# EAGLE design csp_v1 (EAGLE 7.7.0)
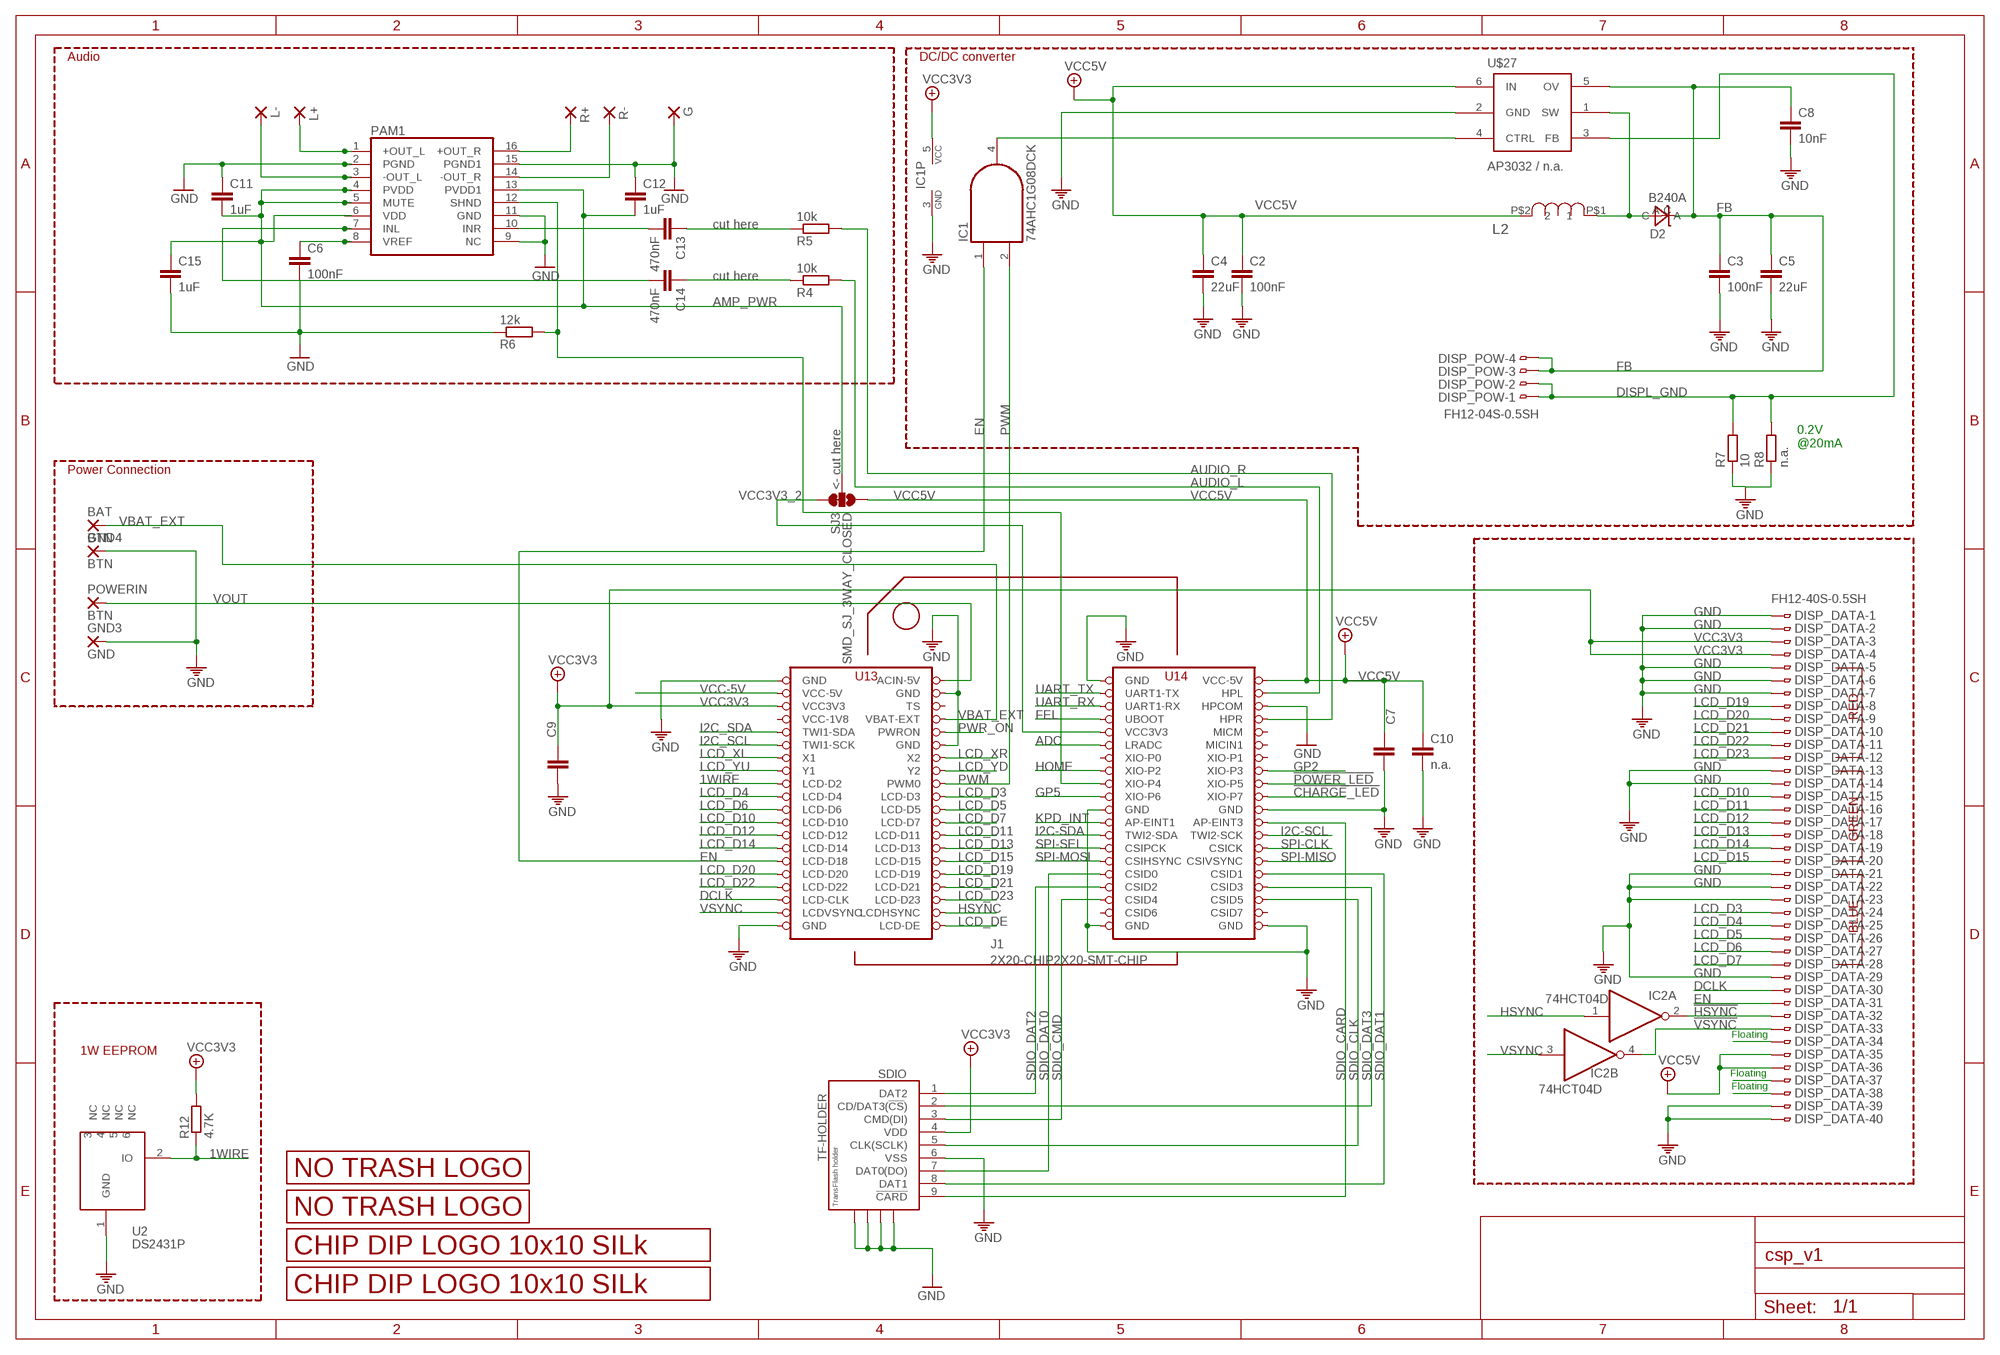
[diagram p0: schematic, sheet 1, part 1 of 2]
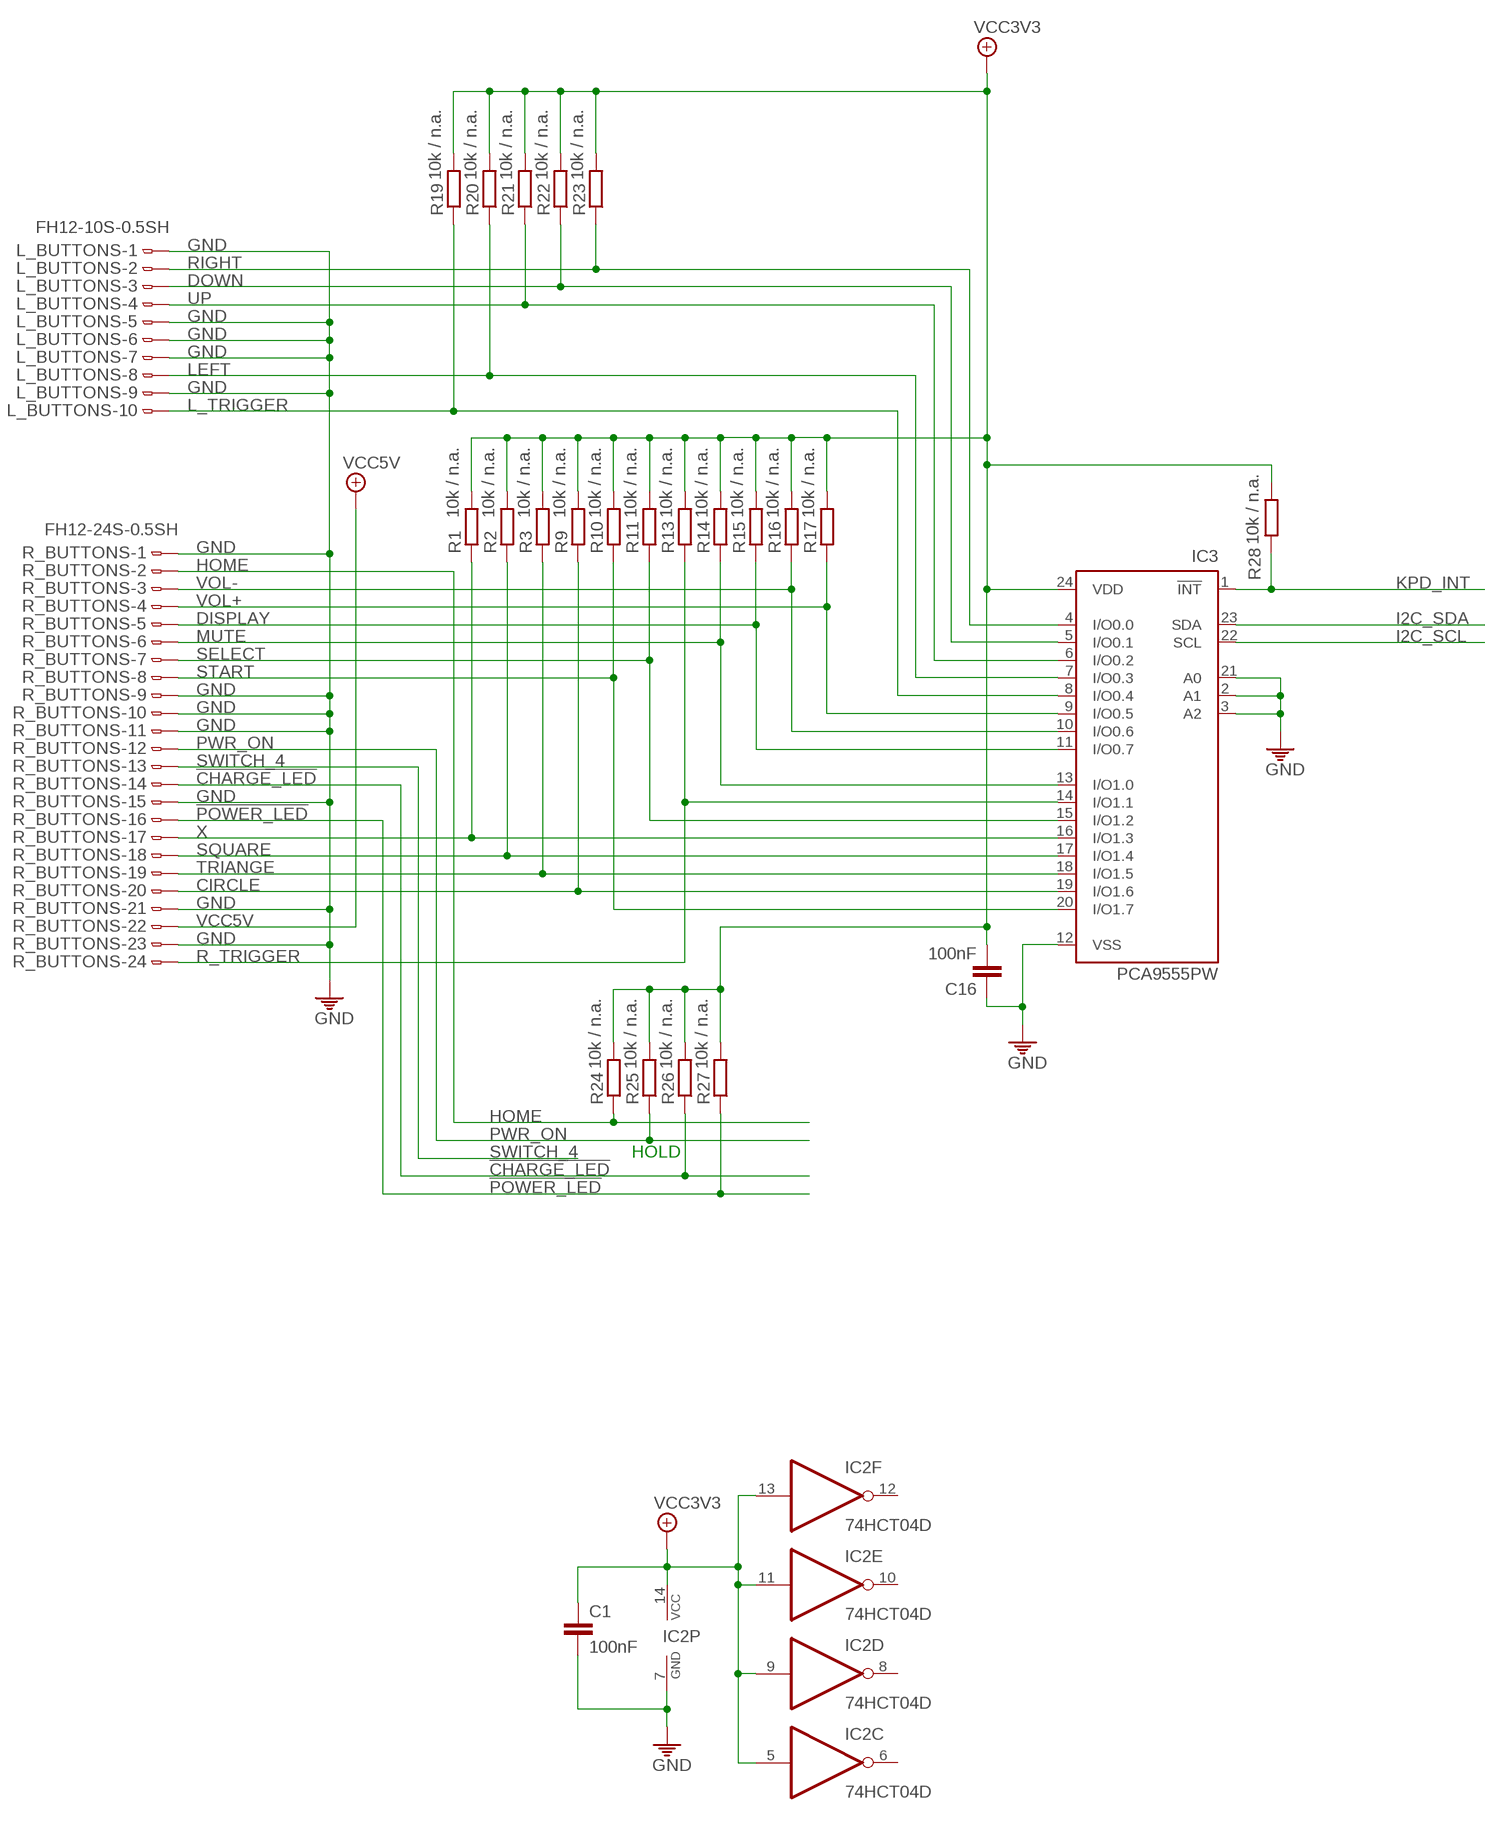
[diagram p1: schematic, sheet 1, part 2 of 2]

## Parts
BAT  BTN  SMD2  [SMD1,27-2,54]
C1  100nF  C-EUC0805  [C0805]
C2  100nF  C-EUC0805  [C0805]
C3  100nF  C-EUC0805  [C0805]
C4  22uF  C-EUC1206  [C1206]
C5  22uF  C-EUC1206  [C1206]
C6  100nF  C-EUC0805  [C0805]
C7  n.a.  C-EUC0805  [C0805]
C8  10nF  C-EUC0805  [C0805]
C9  n.a.  C-EUC0805  [C0805]
C10  n.a.  C-EUC0805  [C0805]
C11  1uF  C-EUC0805  [C0805]
C12  1uF  C-EUC0805  [C0805]
C13  470nF  C-EUC0805  [C0805]
C14  470nF  C-EUC0805  [C0805]
C15  1uF  C-EUC0805  [C0805]
C16  100nF  C-EUC0805  [C0805]
D2  B240A  DIODE_SCHTKY_B240  [DO-214AC]
DISP_DATA  FH12-40S-0.5SH  [FH12-40S-0.5SH]
DISP_POW  FH12-04S-0.5SH  [FH12-04S-0.5SH]
G  1,6/0,8  [1,6/0,8]
GND3  GND  SMD2  [SMD1,27-2,54]
GND4  BTN  SMD2  [SMD1,27-2,54]
IC1  74AHC1G08DCK  [SC70-5]
IC2  74HCT04D  [SO14]
IC3  PCA9555PW  [TSSOP24]
J1  2X20-CHIP2X20-SMT-CHIP  [2XAWHW40_G_SMD_R]
L2  SRN6045-100M  [SRN6045]
L+  1,6/0,8  [1,6/0,8]
L-  1,6/0,8  [1,6/0,8]
L_BUTTONS  FH12-10S-0.5SH  [FH12-10S-0.5SH]
PAM1  PAM8403  [SOP-16]
POWERIN  BTN  SMD2  [SMD1,27-2,54]
R1  10k / n.a.  R-EU_M0805  [M0805]
R2  10k / n.a.  R-EU_M0805  [M0805]
R3  10k / n.a.  R-EU_M0805  [M0805]
R4  10k  R-EU_R0805  [R0805]
R5  10k  R-EU_R0805  [R0805]
R6  12k  R-EU_R0805  [R0805]
R7  10  R-EU_M0805  [M0805]
R8  n.a.  R-EU_M0805  [M0805]
R9  10k / n.a.  R-EU_M0805  [M0805]
R10  10k / n.a.  R-EU_M0805  [M0805]
R11  10k / n.a.  R-EU_M0805  [M0805]
R12  4.7K  R-EU_M0805  [M0805]
R13  10k / n.a.  R-EU_M0805  [M0805]
R14  10k / n.a.  R-EU_M0805  [M0805]
R15  10k / n.a.  R-EU_M0805  [M0805]
R16  10k / n.a.  R-EU_M0805  [M0805]
R17  10k / n.a.  R-EU_M0805  [M0805]
R19  10k / n.a.  R-EU_M0805  [M0805]
R20  10k / n.a.  R-EU_M0805  [M0805]
R21  10k / n.a.  R-EU_M0805  [M0805]
R22  10k / n.a.  R-EU_M0805  [M0805]
R23  10k / n.a.  R-EU_M0805  [M0805]
R24  10k / n.a.  R-EU_M0805  [M0805]
R25  10k / n.a.  R-EU_M0805  [M0805]
R26  10k / n.a.  R-EU_M0805  [M0805]
R27  10k / n.a.  R-EU_M0805  [M0805]
R28  10k / n.a.  R-EU_M0805  [M0805]
R+  1,6/0,8  [1,6/0,8]
R-  1,6/0,8  [1,6/0,8]
R_BUTTONS  FH12-24S-0.5SH  [FH12-24S-0.5SH]
SDIO  TF-HOLDER  [TF-PULL]
SJ3  SMD_SJ_3WAY_CLOSED  [SMD_SJ_3WAY_CLOSED]
U2  DS2431P  [TSOC6]
U$2  LOGO_10X10_SILK  [LOGO2_10X10_SILK]
U$3  LOGO_NO_TRASHROHS  [LOGO_ROHS_SYM]
U$4  LOGO_NO_TRASHNO_TRASH  [LOGO_ROHS_NO_TRASH]
U$5  LOGO_10X10_SILK  [LOGO2_10X10_SILK]
U$27  AP3032 / n.a.  AP3032  [SOT23-6]

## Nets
1WIRE: J1.LCD-D2 R12.1 U2.2(IO)
!CHARGE_LED: J1.XIO-P7 R26.1 R_BUTTONS.14
!HSYNC: DISP_DATA.32 IC2.2(A:O)
!POWER_LED: J1.XIO-P6(XIO-P5) R27.1 R_BUTTONS.16
!VSYNC: DISP_DATA.33 IC2.4(B:O)
ADC: J1.LRADC
AMP_PWR: C11.2 C12.2 C15.1 PAM1.4(PVDD) PAM1.5(MUTE) PAM1.6(VDD) PAM1.13(PVDD1) SJ3.2
AUDIO_L: J1.HPL R4.2
AUDIO_R: J1.HPR R5.2
CIRCLE: IC3.19(I/O1.6) R9.1 R_BUTTONS.20
DCLK: DISP_DATA.30 J1.LCD-CLK
DISPL_GND: DISP_POW.1 DISP_POW.2 R7.2 R8.2 U$27.3(FB)
DISPLAY: IC3.11(I/O0.7) R15.1 R_BUTTONS.5
DOWN: IC3.5(I/O0.1) L_BUTTONS.3 R22.1
EN: DISP_DATA.31 IC1.1(I0) J1.LCD-D18
FB: C3.1 C5.1 C8.1 D2.C DISP_POW.3 DISP_POW.4 U$27.5(OV)
FEL: J1.FEL(UBOOT)
GND: C1.2 C2.2 C3.2 C4.2 C5.2 C6.2 C7.2 C8.2 C9.2 C10.2 C11.1 C12.1 C15.2 C16.1 DISP_DATA.1 DISP_DATA.2 DISP_DATA.5 DISP_DATA.6 DISP_DATA.7 DISP_DATA.13 DISP_DATA.14 DISP_DATA.21 DISP_DATA.22 DISP_DATA.23 DISP_DATA.29 DISP_DATA.39 DISP_DATA.40 G.1(P) GND3.1(P) GND4.1(P) IC1.3(GND) IC2.7(P:GND) IC3.2(A1) IC3.3(A2) IC3.12(VSS) IC3.21(A0) J1.GND@1(GND) J1.GND@2(GND) J1.GND@3(GND) J1.GND@4(GND) J1.GND@5(GND) J1.GND@6(GND) J1.GND@7(GND) J1.GND@8(GND) J1.GND@10(GND) J1.HPCOM L_BUTTONS.1 L_BUTTONS.5 L_BUTTONS.6 L_BUTTONS.7 L_BUTTONS.9 PAM1.2(PGND) PAM1.9(NC) PAM1.11(GND) PAM1.15(PGND1) R6.1 R7.1 R8.1 R_BUTTONS.1 R_BUTTONS.9 R_BUTTONS.10 R_BUTTONS.11 R_BUTTONS.15 R_BUTTONS.21 R_BUTTONS.23 SDIO.6(VSS) SDIO.S1 SDIO.S2 SDIO.S3 SDIO.S4 U2.1(GND) U$27.2(GND)
GP2: J1.XIO-P3
GP3: J1.XIO-P4 PAM1.12(SHND) R6.2
GP5: J1.XIO-P5(XIO-P6)
HOME: J1.XIO-P2 R24.1 R_BUTTONS.2
HSYNC: IC2.1(A:I) J1.LCD-HSYNC(LCDHSYNC)
I2C-SCL: J1.TWI2-SCK
I2C-SDA: J1.TWI2-SDA
I2C_SCL: IC3.22(SCL) J1.TWI1-SCK
I2C_SDA: IC3.23(SDA) J1.TWI1-SDA
INL: C14.2 PAM1.7(INL)
INR: C13.2 PAM1.10(INR)
KPD_INT: IC3.1(!INT) J1.AP-EINT1 R28.1
L+OUT: L+.1(P) PAM1.1(+OUT_L)
L-OUT: L-.1(P) PAM1.3(-OUT_L)
L_TRIGGER: IC3.8(I/O0.4) L_BUTTONS.10 R19.1
LCD_D3: DISP_DATA.24 J1.LCD-D3
LCD_D4: DISP_DATA.25 J1.LCD-D4
LCD_D5: DISP_DATA.26 J1.LCD-D5
LCD_D6: DISP_DATA.27 J1.LCD-D6
LCD_D7: DISP_DATA.28 J1.LCD-D7
LCD_D10: DISP_DATA.15 J1.LCD-D10
LCD_D11: DISP_DATA.16 J1.LCD-D11
LCD_D12: DISP_DATA.17 J1.LCD-D12
LCD_D13: DISP_DATA.18 J1.LCD-D13
LCD_D14: DISP_DATA.19 J1.LCD-D14
LCD_D15: DISP_DATA.20 J1.LCD-D15
LCD_D19: DISP_DATA.8 J1.LCD-D19
LCD_D20: DISP_DATA.9 J1.LCD-D20
LCD_D21: DISP_DATA.10 J1.LCD-D21
LCD_D22: DISP_DATA.11 J1.LCD-D22
LCD_D23: DISP_DATA.12 J1.LCD-D23
LCD_DE: J1.LCD-DE
LCD_XL: J1.X1
LCD_XR: J1.X2
LCD_YD: J1.Y2
LCD_YU: J1.Y1
LEFT: IC3.7(I/O0.3) L_BUTTONS.8 R20.1
MUTE: IC3.13(I/O1.0) R14.1 R_BUTTONS.6
N$1: IC1.4(O) U$27.4(CTRL)
N$9: DISP_DATA.38
N$24: DISP_DATA.37
N$25: DISP_DATA.34
N$38: C6.1 PAM1.8(VREF)
N$41: C14.1 R4.1
N$43: C13.1 R5.1
PWM: IC1.2(I1) J1.PWM0
PWR_ON: J1.PWRON R25.1 R_BUTTONS.12
R+OUT: PAM1.16(+OUT_R) R+.1(P)
R-OUT: PAM1.14(-OUT_R) R-.1(P)
R_TRIGGER: IC3.14(I/O1.1) R13.1 R_BUTTONS.24
RIGHT: IC3.4(I/O0.0) L_BUTTONS.2 R23.1
SDIO_CARD: J1.AP-EINT3 SDIO.9(!CARD)
SDIO_CLK: J1.CSID5 SDIO.5(CLK(SCLK))
SDIO_CMD: J1.CISD4(CSID4) SDIO.3(CMD(DI))
SDIO_DAT0: J1.CSID0 SDIO.7(DAT0(DO))
SDIO_DAT1: J1.CSID1 SDIO.8(DAT1)
SDIO_DAT2: J1.CSID2 SDIO.1(DAT2)
SDIO_DAT3: J1.CSID3 SDIO.2(CD/DAT3(!CS!))
SELECT: IC3.15(I/O1.2) R11.1 R_BUTTONS.7
SPI-CLK: J1.CSICK
SPI-MISO: J1.CSIVSYNC
SPI-MOSI: J1.CSIHYSYNC(CSIHSYNC)
SPI-SEL: J1.CSPICK(CSIPCK)
SQUARE: IC3.17(I/O1.4) R2.1 R_BUTTONS.18
START: IC3.20(I/O1.7) R10.1 R_BUTTONS.8
SWITCH_4: R_BUTTONS.13
TRIANGE: IC3.18(I/O1.5) R3.1 R_BUTTONS.19
UART_RX: J1.UART1-RX
UART_TX: J1.UART1-TX
UP: IC3.6(I/O0.2) L_BUTTONS.4 R21.1
VBAT_EXT: BAT.1(P) J1.BAT(VBAT-EXT)
VCC3V3: C1.1 C9.1 C16.2 DISP_DATA.3 DISP_DATA.4 IC1.5(VCC) IC2.5(C:I) IC2.9(D:I) IC2.11(E:I) IC2.13(F:I) IC2.14(P:VCC) IC3.24(VDD) J1.VCC3V3@2(VCC3V3) R1.2 R2.2 R3.2 R9.2 R10.2 R11.2 R12.2 R13.2 R14.2 R15.2 R16.2 R17.2 R19.2 R20.2 R21.2 R22.2 R23.2 R24.2 R25.2 R26.2 R27.2 R28.2 SDIO.4(VDD)
VCC3V3_2: J1.VCC3V3@1(VCC3V3) SJ3.1
VCC5V: C2.1 C4.1 C7.1 C10.1 DISP_DATA.35 DISP_DATA.36 J1.VCC-5V@2(VCC-5V) L2.P$2 R_BUTTONS.22 SJ3.3 U$27.6(IN)
VCC-5V: J1.VCC-5V@1(VCC-5V)
VOL+: IC3.9(I/O0.5) R17.1 R_BUTTONS.4
VOL-: IC3.10(I/O0.6) R16.1 R_BUTTONS.3
VOUT: J1.CHG-IN(ACIN-5V) POWERIN.1(P)
VREG_OUTPUT: D2.A L2.P$1 U$27.1(SW)
VSYNC: IC2.3(B:I) J1.LCD-VSYNC(LCDVSYNC)
X: IC3.16(I/O1.3) R1.1 R_BUTTONS.17
Unconnected: IC2.6(C:O) IC2.8(D:O) IC2.10(E:O) IC2.12(F:O) J1.CSID6 J1.CSID7 J1.MICIN1 J1.MICM J1.TS J1.XIO-P0 J1.XIO-P1 U2.3(NC) U2.4(NC) U2.5(NC) U2.6(NC)

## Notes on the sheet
- Audio | DC/DC converter
- cut here
- cut here
- <- cut here
- 0.2V
  @20mA
- Power Connection
- RED
- HOLD
- GREEN
- BLUE
- Floating
- 1W EEPROM
- Floating
- Floating

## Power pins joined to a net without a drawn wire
VCC-1V8: J1.VCC1V8(VCC-1V8)

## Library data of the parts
BAT GND3 GND4 POWERIN = wirepad:SMD2: SMD PAD
C1-C16 = rcl:C-EU: CAPACITOR, European symbol
D2 = Keyboard v0_5:DIODE_SCHTKY_B240; DESCRIPTION: DIODE SMD General Purpose 400V 1A 1.4W RoHS DO-214AC; FOOTPRINT: DO-214AC; LINK: http://www.digikey.com/product-detail/en/B240A-13-F/B240A-FDICT-ND/717810; MFG: DIGIKEY; MFG_PN: B240A-FDICT-ND; PART_TYPE: DIODE; PRICE: 0.11; VENDOR: DIODES; VENDOR_PART_NUMBER: B240A-13-F
DISP_DATA = Keyboard v0_5:FH12-40S-0.5S: 0.5mm Pitch Connectors For FPC/FFC Source: Data sheet; DESCRIPTION: CON ffc smd, bottom contact 40pos, 0.50mm R/A; FOOTPRINT: FH12-40S-0.5SH; LINK: http://www.digikey.com/product-detail/en/FH12-40S-0.5SH(55)/HFJ140CT-ND/1110388; MFG: DIGIKEY; MFG_PN: HFJ140CT-ND; VENDOR: HIROSE; VENDOR_PART_NUMBER: FH12-40S-0.5SH(55)
DISP_POW = JKW_CHIP:FH12-04S-0.5S: 0.5mm Pitch Connectors For FPC/FFC Source: Data sheet; MPN: FH12-10S-0.5SH(55); OC_FARNELL: 1324540; OC_NEWARK: 34M6152
G L+ L- R+ R- = wirepad:1,6/0,8: THROUGH-HOLE PAD
IC1 = 74xx-little-us:74*1G08: 2-input AND gate
IC2 = JKW_CHIP:74*04: Hex INVERTER
IC3 = micro-philips:PCA9555: 16-bit I2C and SMBus I/O port with interrupt Source: PCA9555_5.pdf; MPN: PCA9555PW; OC_FARNELL: 1408297; OC_NEWARK: 63K6069
J1 = JKW_CHIP:2X20-CHIP: Chip header
L2 = Keyboard v0_5:SRN6045-100M; DESCRIPTION: power inductor 10uH 2.5A 58.6 mohm; FOOTPRINT: SRN6045; LINK: http://www.digikey.com/product-detail/en/SRN6045-100M/SRN6045-100MTR-ND/2756120; MFG: DIGIKEY; MFG_PN: SRN6045-100MTR-ND; PART_TYPE: IND; PRICE: 0.15; TOLLERANCE: ±20%; VENDOR: BOURNS; VENDOR_PART_NUMBER: SRN6045-100M
L_BUTTONS = con-hirose:FH12-10S-0.5S: 0.5mm Pitch Connectors For FPC/FFC Source: Data sheet; MPN: FH12-10S-0.5SH(55); OC_FARNELL: 1324540; OC_NEWARK: 34M6152
PAM1 = JKW_CHIP:PAM8403: Dual channel audio amplifier IC - PAM8403
R1-R17 R19-R28 = rcl:R-EU_: RESISTOR, European symbol
R_BUTTONS = con-hirose:FH12-24S-0.5S: 0.5mm Pitch Connectors For FPC/FFC Source: Data sheet; MPN: FH12-24S-0.5SH(55); OC_FARNELL: 1324552; OC_NEWARK: 34M6170
SDIO = JKW_CHIP:TF-HOLDER: TF / Micro SD socket is PUSH-PUSH type, the card can be pushed into and auto locked and pushed out by simply press the card. Surface Mounting type.
SJ3 = JKW_CHIP:SMD_SJ_3WAY_CLOSED
U2 = JKW_CHIP:DS2431: 1024-Bit EEPROM This chip provides a 4x256 Bit EEPROM, which can be programmed@5V. Write protection and OTP emulation are available, too. Author: Jan Kandziora <jjj@gmx.de>; DESCRIPTION: IC, 1024-Bit, 1-Wire EEPROM, TSOC6; FOOTPRINT: TSOC6; LINK: http://www.digikey.com/product-detail/en/DS2431P%2BT%26R/DS2431P%2BT%26RCT-ND/3647900; MFG: DIGIKEY; MFG_PN: DS2431P+T&RCT-ND; PART_TYPE: IC; PRICE: 0.98; VENDOR: MAXIM; VENDOR_PART_NUMBER: DS2431P+T&R
U$2 U$5 = JKW_CHIP:LOGO_10X10_SILK
U$3 U$4 = JKW_CHIP:LOGO_NO_TRASH
U$27 = JKW_CHIP:AP3032

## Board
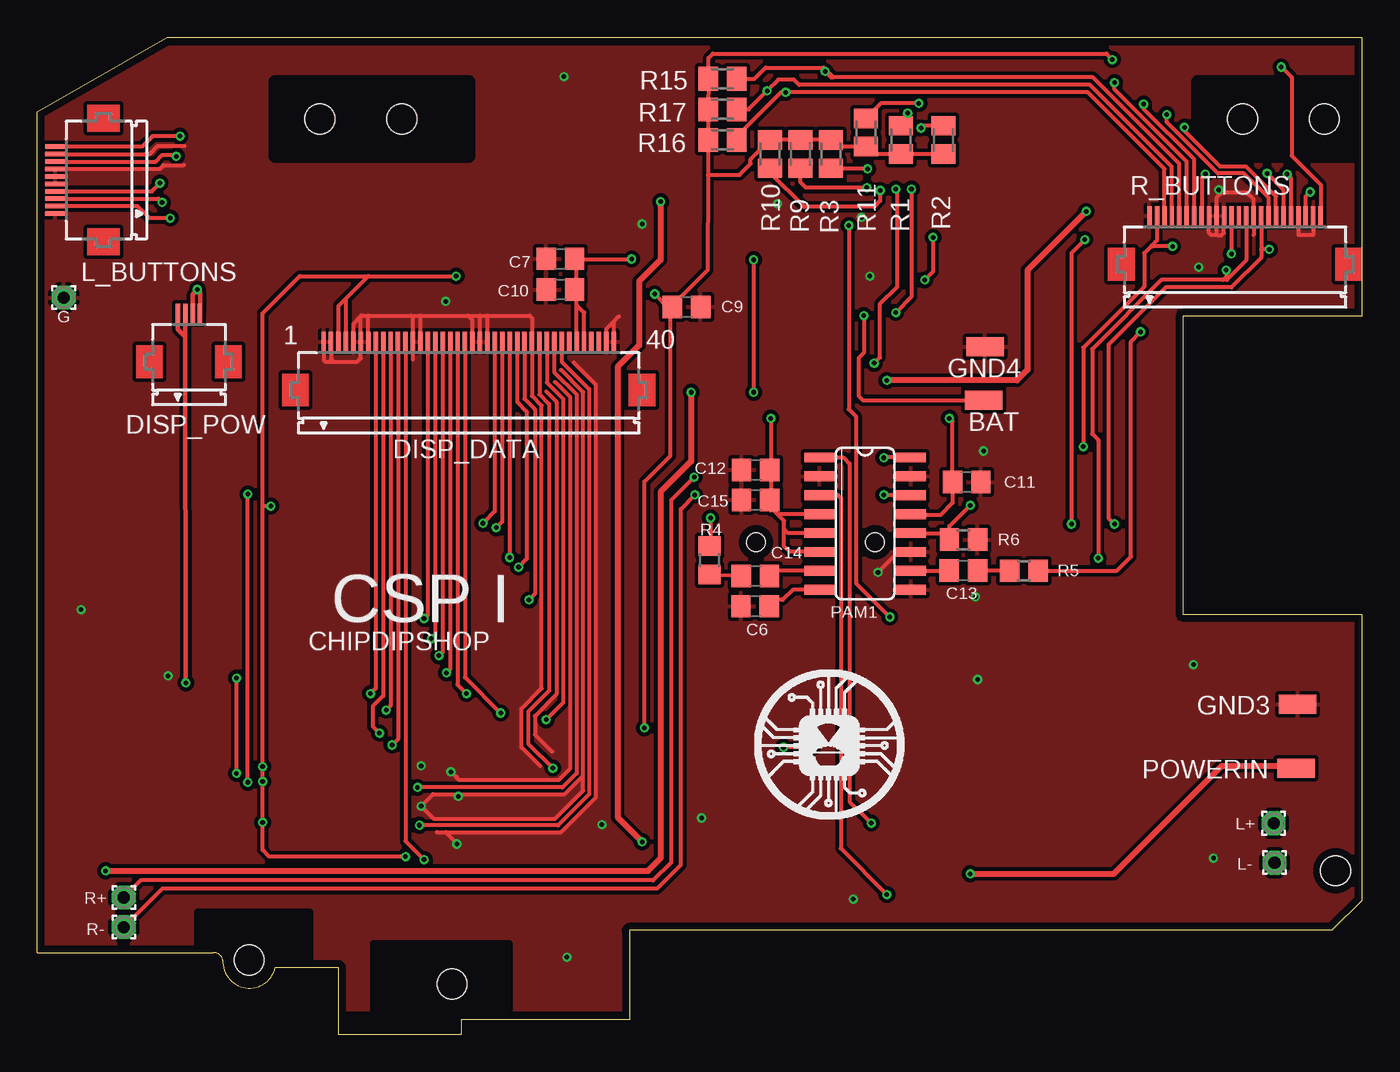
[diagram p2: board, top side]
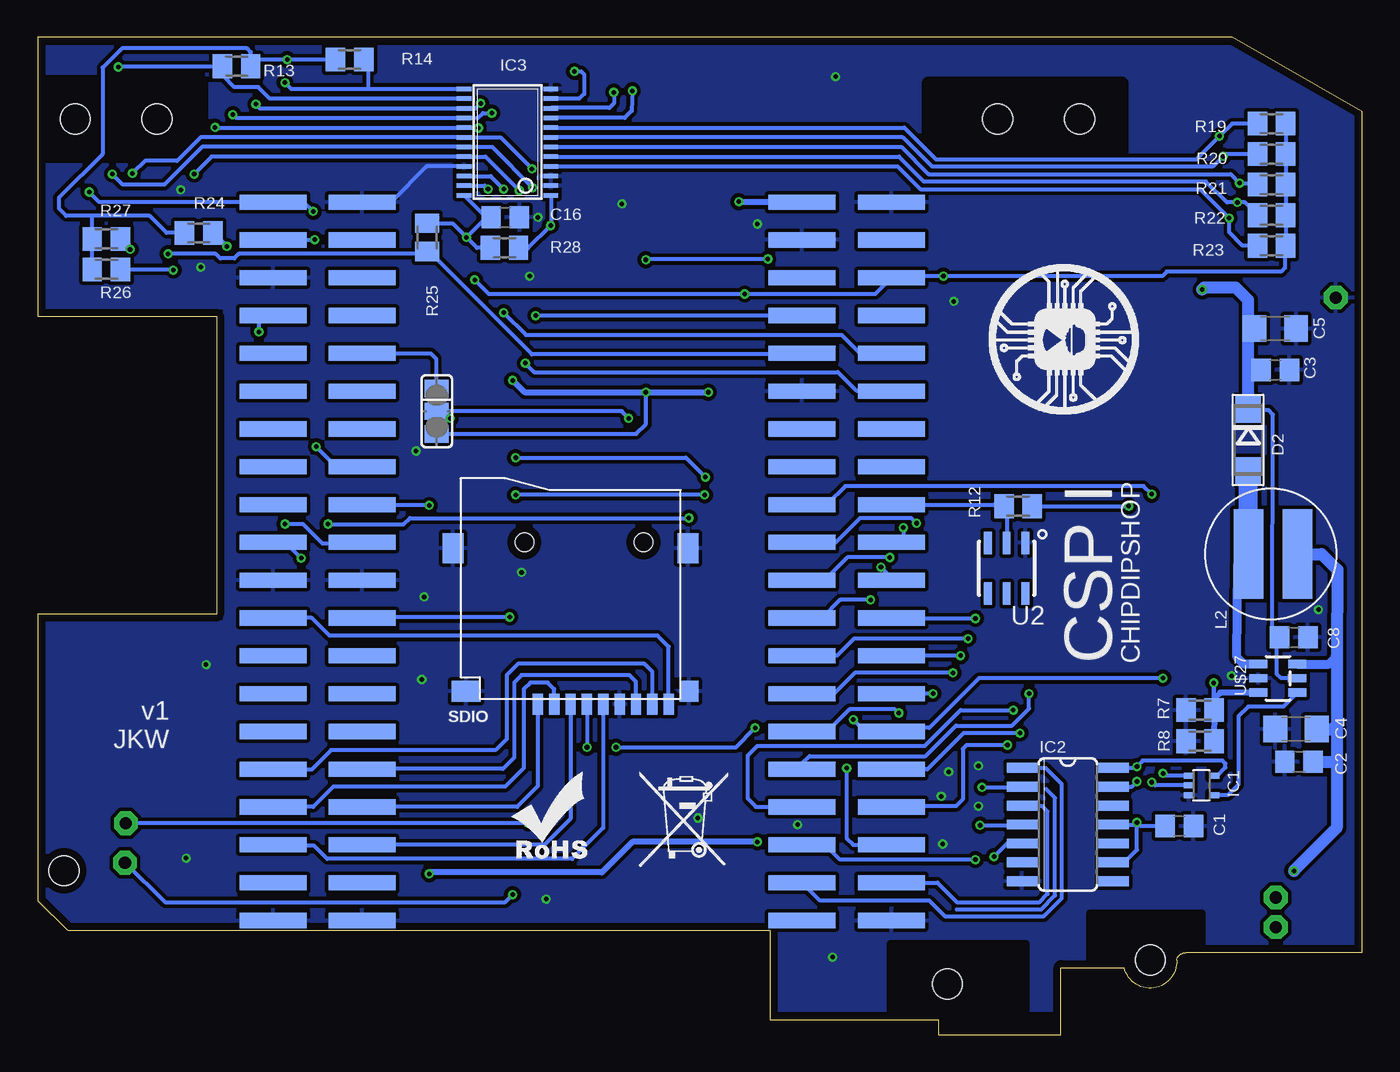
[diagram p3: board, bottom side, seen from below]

Size 89 x 67 mm. Coordinates in mm from the lower left corner, seen from the top.
Outline: 39.8,1 28.5,1 28.5,0 20.25,0 20.25,4.5 16,4.5 arc-170 12.47,5 arc80 11.85,5.5 0,5.5 0,62 8.75,67 89,67 89,48.25 77,48.25 77,28.25 89,28.25 89,9 87,7 39.8,7 39.8,1
Copper layers (1*16): Top 0.035mm / dielectric 1.6mm / Bottom 0.035mm
Design rules "Elecrow_2-layer_PCB_eagle_rule": minimum track width 6mil, minimum drill 12mil, track to track 6mil, track to pad 6mil, pad to pad 6mil, via to via 8mil, smd to smd 0mil, copper to edge 20mil, drill to drill 10mil, minimum pad ring 6mil, minimum via ring 6mil, stop-mask expansion 0mil, vias tented up to drill 100mil, thermal gap 10mil
Holes 2 mm at 27.88,3.39 14.25,5 19,61.5 86.5,61.5 81,61.5 24.5,61.5 87.25,11
bKeepout: area 14.4,3.2 to 20.6,65.1
tRestrict: area 16,59 to 29,64; area 78,59 to 88.6,64; area 22.6,1.3 to 31.7,6.1; area 10.8,2.9 to 18.3,8.2
bRestrict: area 16.1,58.9 to 29.1,63.9; area 78,59 to 88.6,64; area 10.8,2.8 to 18.3,8.2; area 22.6,1.3 to 31.7,6.1

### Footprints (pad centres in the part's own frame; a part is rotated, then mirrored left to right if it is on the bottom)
SMD1,27-2,54 = smd 1.27 x 2.54: 1 0,0
C0805 = smd 1.3 x 1.5: 1 -0.95,0; 2 0.95,0
C1206 = smd 1.6 x 1.8: 1 -1.4,0; 2 1.4,0
DO-214AC = smd 1.8 x 1.7: A 2.05,0; C -2.05,0
FH12-40S-0.5SH = smd 0.3 x 1.3: 1 -9.75,3.25; 2 -9.25,3.25; 3 -8.75,3.25; 4 -8.25,3.25; 5 -7.75,3.25; 6 -7.25,3.25; 7 -6.75,3.25; 8 -6.25,3.25; 9 -5.75,3.25; 10 -5.25,3.25; 11 -4.75,3.25; 12 -4.25,3.25; 13 -3.75,3.25; 14 -3.25,3.25; 15 -2.75,3.25; 16 -2.25,3.25; 17 -1.75,3.25; 18 -1.25,3.25; 19 -0.75,3.25; 20 -0.25,3.25; 21 0.25,3.25; 22 0.75,3.25; 23 1.25,3.25; 24 1.75,3.25; 25 2.25,3.25; 26 2.75,3.25; 27 3.25,3.25; 28 3.75,3.25; 29 4.25,3.25; 30 4.75,3.25; 31 5.25,3.25; 32 5.75,3.25; 33 6.25,3.25; 34 6.75,3.25; 35 7.25,3.25; 36 7.75,3.25; 37 8.25,3.25; 38 8.75,3.25; 39 9.25,3.25; 40 9.75,3.25
FH12-04S-0.5SH = smd 0.3 x 1.3: 1 -0.75,3.25; 2 -0.25,3.25; 3 0.25,3.25; 4 0.75,3.25
1,6/0,8 = drill 0.813 pad 1.6 octagon: 1 0,0
SC70-5 = smd 0.4 x 0.7: 1 -0.65,-0.85; 2 0,-0.85; 3 0.65,-0.85; 4 0.65,0.85; 5 -0.65,0.85
SO14 = smd 0.66 x 2.032: 1 -3.81,-3.073; 2 -2.54,-3.073; 3 -1.27,-3.073; 4 0,-3.073; 5 1.27,-3.073; 6 2.54,-3.073; 7 3.81,-3.073; 8 3.81,3.073; 9 2.54,3.073; 10 1.27,3.073; 11 0,3.073; 12 -1.27,3.073; 13 -2.54,3.073; 14 -3.81,3.073
TSSOP24 = smd 0.305 x 0.991: 1 -3.575,-2.918; 2 -2.925,-2.918; 3 -2.275,-2.918; 4 -1.625,-2.918; 5 -0.975,-2.918; 6 -0.325,-2.918; 7 0.325,-2.918; 8 0.975,-2.918; 9 1.625,-2.918; 10 2.275,-2.918; 11 2.925,-2.918; 12 3.575,-2.918; 13 3.575,2.918; 14 2.925,2.918; 15 2.275,2.918; 16 1.625,2.918; 17 0.975,2.918; 18 0.325,2.918; 19 -0.325,2.918; 20 -0.975,2.918; 21 -1.625,2.918; 22 -2.275,2.918; 23 -2.925,2.918; 24 -3.575,2.918
2XAWHW40_G_SMD_R = smd 4.5 x 1.02 bottom: AP-EINT1 35.1,21.59; AP-EINT3 41.1,21.59; BAT 5.54,41.91; CHG-IN 5.54,49.53; CISD4 35.1,6.35; CSICK 41.1,16.51; CSID0 35.1,11.43; CSID1 41.1,11.43; CSID2 35.1,8.89; CSID3 41.1,8.89; CSID5 41.1,6.35; CSID6 35.1,3.81; CSID7 41.1,3.81; CSIHYSYNC 35.1,13.97; CSIVSYNC 41.1,13.97; CSPICK 35.1,16.51; FEL 35.1,41.91; GND@1 -0.46,49.53; GND@2 5.54,46.99; GND@3 5.54,36.83; GND@4 -0.46,1.27; GND@5 41.1,1.27; GND@6 35.1,1.27; GND@7 41.1,24.13; GND@8 35.1,24.13; GND@10 35.1,49.53; HPCOM 41.1,44.45; HPL 41.1,46.99; HPR 41.1,41.91; LCD-CLK -0.46,6.35; LCD-D2 -0.46,29.21; LCD-D3 5.54,26.67; LCD-D4 -0.46,26.67; LCD-D5 5.54,24.13; LCD-D6 -0.46,24.13; LCD-D7 5.54,21.59; LCD-D10 -0.46,21.59; LCD-D11 5.54,19.05; LCD-D12 -0.46,19.05; LCD-D13 5.54,16.51; LCD-D14 -0.46,16.51; LCD-D15 5.54,13.97; LCD-D18 -0.46,13.97; LCD-D19 5.54,11.43; LCD-D20 -0.46,11.43; LCD-D21 5.54,8.89; LCD-D22 -0.46,8.89; LCD-D23 5.54,6.35; LCD-DE 5.54,1.27; LCD-HSYNC 5.54,3.81; LCD-VSYNC -0.46,3.81; LRADC 35.1,36.83; MICIN1 41.1,36.83; MICM 41.1,39.37; PWM0 5.54,29.21; PWRON 5.54,39.37; TS 5.54,44.45; TWI1-SCK -0.46,36.83; TWI1-SDA -0.46,39.37; TWI2-SCK 41.1,19.05; TWI2-SDA 35.1,19.05; UART1-RX 35.1,44.45; UART1-TX 35.1,46.99; VCC1V8 -0.46,41.91; VCC3V3@1 35.1,39.37; VCC3V3@2 -0.46,44.45; VCC-5V@1 -0.46,46.99; VCC-5V@2 41.1,49.53; X1 -0.46,34.29; X2 5.54,34.29; XIO-P0 35.1,34.29; XIO-P1 41.1,34.29; XIO-P2 35.1,31.75; XIO-P3 41.1,31.75; XIO-P4 35.1,29.21; XIO-P5 41.1,29.21; XIO-P6 35.1,26.67; XIO-P7 41.1,26.67; Y1 -0.46,31.75; Y2 5.54,31.75
SRN6045 = smd 2 x 6: P$1 1.5,0; P$2 -1.8,0
FH12-10S-0.5SH = smd 0.3 x 1.3: 1 -2.25,3.25; 2 -1.75,3.25; 3 -1.25,3.25; 4 -0.75,3.25; 5 -0.25,3.25; 6 0.25,3.25; 7 0.75,3.25; 8 1.25,3.25; 9 1.75,3.25; 10 2.25,3.25
SOP-16 = smd 0.66 x 2.032: 1 -4.445,-3.073; 2 -3.175,-3.073; 3 -1.905,-3.073; 4 -0.635,-3.073; 5 0.635,-3.073; 6 1.905,-3.073; 7 3.175,-3.073; 8 4.445,-3.073; 9 4.445,3.073; 10 3.175,3.073; 11 1.905,3.073; 12 0.635,3.073; 13 -0.635,3.073; 14 -1.905,3.073; 15 -3.175,3.073; 16 -4.445,3.073
M0805 = smd 1.3 x 1.6: 1 -0.95,0; 2 0.95,0
R0805 = smd 1.3 x 1.5: 1 -0.95,0; 2 0.95,0
FH12-24S-0.5SH = smd 0.3 x 1.3: 1 -5.75,3.25; 2 -5.25,3.25; 3 -4.75,3.25; 4 -4.25,3.25; 5 -3.75,3.25; 6 -3.25,3.25; 7 -2.75,3.25; 8 -2.25,3.25; 9 -1.75,3.25; 10 -1.25,3.25; 11 -0.75,3.25; 12 -0.25,3.25; 13 0.25,3.25; 14 0.75,3.25; 15 1.25,3.25; 16 1.75,3.25; 17 2.25,3.25; 18 2.75,3.25; 19 3.25,3.25; 20 3.75,3.25; 21 4.25,3.25; 22 4.75,3.25; 23 5.25,3.25; 24 5.75,3.25
TF-PULL = smd 0.7 x 1.4: 1 -2.2,-7.62; 2 -1.1,-7.62; 3 0,-7.62; 4 1.1,-7.62; 5 2.2,-7.62; 6 3.3,-7.62; 7 4.4,-7.62; 8 5.5,-7.62; 9 6.6,-7.62 | smd 1.4 x 2: S1 -7.9,2.85; S2 7.9,2.85 | smd 1.28 x 1.4: S3 7.96,-6.75 | smd 1.95 x 1.4: S4 -7.025,-6.75 | hole 1.25: -3.1,3.25; 4.9,3.25
SMD_SJ_3WAY_CLOSED = smd 1.168 x 1.6: 1 -1.524,0; 2 0,0; 3 1.524,0
TSOC6 = smd 0.53 x 1.53: 1 -1.27,-1.7; 2 0,-1.7; 3 1.27,-1.7; 4 1.27,1.7; 5 0,1.7; 6 -1.27,1.7
SOT23-6 = smd 0.559 x 1.219: 1 -0.95,-1.3; 2 0,-1.3; 3 0.965,-1.3; 4 0.965,1.321; 5 0,1.3; 6 -0.95,1.321

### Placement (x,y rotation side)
BAT  63.6,42.6 90 top
C1  12.3,14 0 bottom
C2  4.26,18.32 180 bottom
C3  5.85,44.65 0 bottom
C4  4.45,20.52 180 bottom
C5  5.85,47.43 0 bottom
C6  48.25,28.78 180 top
C7  35.16,52.11 180 top
C8  4.6,26.68 0 bottom
C9  43.63,48.88 0 top
C10  35.16,50.05 180 top
C11  62.47,37.11 180 top
C12  48.28,37.93 0 top
C13  62.24,31.18 180 top
C14  48.26,30.81 0 top
C15  48.28,35.91 180 top
C16  57.6,54.9 180 bottom
D2  7.68,39.95 270 bottom
DISP_DATA  29,43.3 0 top
DISP_POW  10.2,45.2 0 top
G  1.78,49.51 0 top
GND3  84.7,22.2 90 top
GND4  63.7,46.2 90 top
IC1  10.81,16.74 270 bottom
IC2  19.79,14.11 270 bottom
IC3  57.45,59.95 90 bottom
J1  32.1,6.39 0 top
L2  6.15,32.28 180 bottom
L+  83.09,14.2 0 top
L-  83.15,11.55 0 top
L_BUTTONS  4.45,57.4 90 top
PAM1  55.64,34.33 270 top
POWERIN  84.6,17.9 90 top
R1  58.05,60.1 270 top
R2  60.9,60.1 270 top
R3  53.35,59.15 90 top
R4  45.18,31.86 90 top
R5  66.31,31.16 0 top
R6  62.25,33.25 180 top
R7  10.9,21.8 0 bottom
R8  10.9,19.7 0 bottom
R9  51.3,59.15 90 top
R10  49.25,59.15 90 top
R11  55.7,60.6 270 top
R12  23.13,35.5 0 bottom
R13  75.65,65.05 0 bottom
R14  68.05,65.5 180 bottom
R15  46.05,64.2 180 top
R16  46.05,60.1 180 top
R17  46.05,62.15 180 top
R19  6.1,61.2 0 bottom
R20  6.1,59.15 0 bottom
R21  6.1,57.1 0 bottom
R22  6.1,55.05 0 bottom
R23  6.1,53 0 bottom
R24  78.2,53.85 180 bottom
R25  62.85,53.55 90 bottom
R26  84.4,51.4 180 bottom
R27  84.4,53.45 180 bottom
R28  57.65,52.85 180 bottom
R+  5.82,9.21 0 top
R-  5.82,7.22 0 top
R_BUTTONS  80.5,51.75 0 top
SDIO  53.21,29.82 0 bottom
SJ3  62.2,41.88 270 bottom
U2  23.9,31.33 180 bottom
U$2  48.2,14.46 0 top
U$3  57.63,11.76 0 bottom
U$4  48.62,11.27 0 bottom
U$5  15.04,41.68 90 bottom
U$27  5.68,23.94 270 bottom

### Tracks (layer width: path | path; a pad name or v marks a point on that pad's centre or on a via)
1WIRE
  Bottom 0.254: J1.LCD-D2 24.75,35.6 24.2,35.05 | 24.2,35.05 23.9,34.75 23.9,33.53 U2.2 | R12.1 24.08,35.17 24.2,35.05
!CHARGE_LED  (via drill 0.3)
  Top 0.254: R_BUTTONS.14 81.25,52 79.95,50.7 79.7,50.7 | 79.7,50.7 75.55,50.7 70.9,46.05 70.9,40.35 71.3,39.95 v71.3,32 | v79.9,51.35 79.9,50.9 79.7,50.7
  Bottom 0.254: J1.XIO-P7 73.11,33.15 72.45,33.15 72.55,33.05 72.35,33.05 v71.3,32 | R26.1 79.95,51.4 v79.9,51.35
!HSYNC  (via drill 0.3)
  Top 0.254: DISP_DATA.32 34.75,44.5 36.25,43 36.25,17.55 35.3,16.6 v25.55,16.6
  Bottom 0.254: v25.55,16.6 22.91,16.6 IC2.2
!POWER_LED  (via drill 0.3)
  Top 0.254: R_BUTTONS.16 82.25,52.75 | 82.25,52.75 82.25,52.2 80.25,50.2 75.85,50.2 72,46.35 72,34.7 v72.4,34.3 | v82.8,52.75 82.25,52.75
  Bottom 0.254: v72.4,34.3 71.2,34.3 69.9,33 67.26,33 J1.XIO-P6 | R27.1 v82.8,52.75
!VSYNC  (via drill 0.3)
  Top 0.254: DISP_DATA.33 35.25,45.21 37.1,43.36 37.1,16.15 35.01,14.06 v25.69,14.06
  Bottom 0.254: v25.69,14.06 22.91,14.06 IC2.4
AMP_PWR  (via drill 0.3)
  Top 0.254: PAM1.13 58.77,34.9 60.7,34.9 61.52,35.72 C11.2 61.52,41.18 v61.3,41.4 | v49.3,41.4 49.3,37.9 | 49.3,37.9 49.3,35.9 | 49.3,35.9 49.3,35.4 | 49.3,35.4 49.3,35.2 | 52.65,34.95 52.64,34.96 PAM1.4 49.74,34.96 | PAM1.5 50.46,33.69 50.2,33.95 | 50.2,33.95 50.2,34.5 49.74,34.96 | PAM1.6 50.58,32.42 50.2,32.8 50.2,33.95 | 49.74,34.96 49.3,35.4 | C15.1 49.29,35.91 49.3,35.9 | C12.2 49.27,37.93 49.3,37.9
  Bottom 0.254: v49.3,41.4 49.77,41.88 SJ3.2 61.73,41.4 v61.3,41.4
AUDIO_L  (via drill 0.3)
  Top 0.254: v70.4,53.4 69.5,52.5 v69.5,34.3 | v45.25,34.7 45.25,32.88 R4.2
  Bottom 0.254: J1.HPL 70.42,53.38 v70.4,53.4 | v69.5,34.3 69.45,34.25 64.45,34.25 64,34.7 v45.25,34.7
AUDIO_R  (via drill 0.3)
  Top 0.254: R5.2 72.56,31.16 73.5,32.1 73.5,46.55 v74.15,47.2
  Bottom 0.254: v74.15,47.2 74.15,47.8 73.75,48.2 73.3,48.2 J1.HPR
CIRCLE  (via drill 0.3)
  Top 0.254: v84,57.8 84.25,57.55 R_BUTTONS.20 | v55.75,56.9 51.65,56.9 51.3,57.25 R9.1
  Bottom 0.254: v84,57.8 83.3,57.1 80.5,57.1 77.97,59.62 IC3.19 58.48,59.62 v55.75,56.9
DCLK  (via drill 0.3)
  Top 0.254: DISP_DATA.30 33.75,43 34.4,42.35 34.4,23.1 33,21.7 33,19.55 v34.65,17.9
  Bottom 0.254: v34.65,17.9 34.65,13.2 34.2,12.75 J1.LCD-CLK
DISPL_GND  (via drill 0.3)
  Top 0.305: DISP_POW.2 9.95,46.89 | 9.95,46.89 v9.99,23.63 | DISP_POW.1 9.45,47.39 9.95,46.89
  Bottom 0.305: v9.99,23.63 9.99,21.64 R7.2
  Bottom 0.406: U$27.3 9.54,22.98 9.91,22.61 9.91,21.71 R7.2 9.98,19.79 R8.2
DISPLAY  (via drill 0.3)
  Top 0.254: R_BUTTONS.5 76.75,58.5 70.95,64.3 53.5,64.3 | 53.5,64.3 53.35,64.3 v52.95,64.7 | R15.1 48.2,64.2 48.95,64.95 52.85,64.95 53.5,64.3
  Bottom 0.254: v52.95,64.7 52.5,64.7 52.3,64.5 52.3,63.2 52.62,62.88 IC3.11
DOWN  (via drill 0.3)
  Top 0.254: L_BUTTONS.3 8.15,56.15 v8.4,55.9
  Bottom 0.254: IC3.5 31.12,58.98 29.45,57.3 10.5,57.3 9.1,55.9 v8.4,55.9 7.9,55.9 R22.1
EN  (via drill 0.3)
  Top 0.254: DISP_DATA.31 34.25,43.8 35.35,42.7 35.35,22.3 v34.2,21.15 | v13.4,17.55 v13.4,23.95
  Bottom 0.254: v34.2,21.15 33.41,20.36 J1.LCD-D18 31.4,20.6 29.1,20.6 25.75,23.95 v13.4,23.95 | IC1.1 13.24,17.39 v13.4,17.55
FB  (via drill 0.3)
  Top 0.305: DISP_POW.4 10.95,49.86 v10.76,50.05 10.45,49.74 DISP_POW.3
  Bottom 0.254: U$27.5 5.45,23.94 5.73,24.22 5.73,26.59 6.05,26.91 6.01,41.64 6.3,41.93 7.61,41.93 D2.C | C5.1 7.65,47.43 7.68,47.45 | C3.1 6.8,44.75 7.68,44.75
  Bottom 0.813: D2.C 7.68,44.75 7.68,47.45 7.68,49.34 8.51,50.17 10.64,50.17 v10.76,50.05 | C8.1 5.64,26.59 5.73,26.59
GND  (via drill 0.3)
  Top 0.254: DISP_DATA.40 38.75,47.91 | 38.75,47.91 39.08,48.24 | DISP_DATA.39 38.25,47.41 38.75,47.91 | 27.45,13.6 35.2,13.6 37.55,15.95 37.55,43.65 36.05,45.15 | 36.65,17.35 35.45,16.15 26.6,16.15 v25.8,15.35 26.68,14.47 34.77,14.47 36.69,16.39 36.69,43.16 35.2,44.65 | 34.2,43.2 34.9,42.5 34.9,22.85 33.45,21.4 33.45,20.15 34.6,19 | 33.8,18.05 32.55,19.3 32.55,21.9 33.9,23.25 33.9,42.25 33.25,42.9 DISP_DATA.29 33.25,48.15 33.1,48.3 30.25,48.3 | DISP_DATA.5 21.25,47.75 21.75,48.25 | DISP_DATA.6 21.75,48.25 | 21.75,48.25 21.8,48.3 | DISP_DATA.6 21.75,48.2 21.85,48.3 22.25,48.3 | 22.25,48.3 25.1,48.3 | 25.1,48.3 25.75,48.3 | 25.75,48.3 28.95,48.3 | 28.95,48.3 29.75,48.3 | 29.75,48.3 30.25,48.3 | DISP_DATA.23 30.25,48.3 | DISP_DATA.22 29.75,48.3 | DISP_DATA.21 29.25,48 28.95,48.3 | DISP_DATA.14 25.75,48.3 | 25.1,48.3 25.25,48.15 DISP_DATA.13 25.25,45.35 | DISP_DATA.7 22.25,48.3 | DISP_DATA.2 19.75,45.35 19.9,45.2 | 19.9,45.2 21.5,45.2 21.75,45.45 DISP_DATA.6 | DISP_DATA.1 19.25,45.3 19.35,45.2 19.9,45.2 | R_BUTTONS.23 85.75,53.7 84.75,53.7 R_BUTTONS.21 | 79.3,53.7 78.9,53.7 78.75,53.85 R_BUTTONS.9 | 79.3,53.7 79.25,53.75 R_BUTTONS.10 79.25,56.2 79.6,56.55 | 81.75,53.7 R_BUTTONS.15 81.75,56.1 81.3,56.55 79.6,56.55 | 79.3,53.7 79.6,53.7 79.75,53.85 R_BUTTONS.11 | L_BUTTONS.9 7.55,59.15 8.1,59.7 9.9,59.7 | L_BUTTONS.7 8.25,58.15 8.5,58.4 9.85,58.4 | 26.85,13.6 27.45,13.6 | 27.45,13.6 28.2,12.85 | 79.6,56.55 v79.4,56.75 | PAM1.11 57.87,32.42 v56.5,31.05 | 34.8,43.85 35.8,42.85 35.8,17.85 35.05,17.1 28.35,17.1 28.2,17.25 28.2,17.3 27.85,17.65
  Bottom 0.254: IC3.21 62.88,58.33 65.28,55.92 J1.GND@10
  other vias: 40.65,54.45 27.45,49.25 63.6,39.2 63.05,29.4 63.2,23.85 54.85,9.1 79.05,11.85 77.7,24.85 28.2,12.8 25.8,18.05 27.8,17.65 8.8,24.1 2.95,28.55 78.05,51.55 49.75,55.8 55.95,50.95 55.4,54.9 35.4,64.35 28.3,16 37.95,14.1 44.65,14.55 35.6,5.2
  pour Bottom (isolate 0.254): 0.45,61.55 8.8,66.4 88.6,66.4 88.6,63.9 88.6,48.85 79.4,48.85 76.45,48.85 76.45,47.05 76.45,27.7 88.45,27.7 88.45,9.2 86.75,7.5 39.5,7.5 39.5,1.65 20.7,1.65 20.7,4.75 13.15,4.75 13.15,5.85 0.45,5.85 0.45,6.65
  pour Top (isolate 0.254): 0.45,61.55 8.8,66.4 88.6,66.4 88.6,63.9 88.6,48.85 79.4,48.85 76.45,48.85 76.45,47.05 76.45,27.7 88.45,27.7 88.45,9.2 86.75,7.5 39.5,7.5 39.5,1.65 20.7,1.65 20.7,4.75 13.15,4.75 13.15,5.85 0.45,5.85 0.45,6.65
GP3  (via drill 0.3)
  Top 0.254: PAM1.12 60.86,33.69 R6.2 61.3,34.15 v62.7,35.55
  Bottom 0.254: v62.7,35.55 67.15,35.55 J1.XIO-P4
HOME  (via drill 0.3)
  Top 0.254: R_BUTTONS.2 75.25,53.35 74.9,53 | 74.9,53 74.4,52.5 74.4,50.25 70.3,46.15 v70.3,39.5 | v76.3,52.95 74.95,52.95 74.9,53
  Bottom 0.254: J1.XIO-P2 68.95,38.15 v70.3,39.5 | R24.1 77.2,53.85 v76.3,52.95
HSYNC
  Bottom 0.254: IC2.1 21.3,17.92 20.2,16.82 20.2,9.15 21.4,7.95 28.05,7.95 29.1,9 36.44,9 J1.LCD-HSYNC
I2C_SCL  (via drill 0.3)
  Top 0.254: v56.25,45.1 56.65,45.5 56.65,49.1 57.8,50.25 57.8,56.7 v57.7,56.8
  Bottom 0.254: v56.25,45.1 55.65,44.5 35.25,44.5 34,43.25 31.67,43.25 J1.TWI1-SCK | IC3.22 58.58,57.67 v57.7,56.8
I2C_SDA  (via drill 0.3)
  Top 0.254: v58.75,56.8 58.75,49.55 v57.7,48.5
  Bottom 0.254: IC3.23 58.98,57.02 v58.75,56.8 | v57.7,48.5 56.2,47 35,47 33.76,45.76 J1.TWI1-SDA
INL
  Top 0.254: PAM1.7 49.27,31.15 C14.2
INR
  Top 0.254: PAM1.10 61.26,31.15 C13.2
KPD_INT  (via drill 0.3)
  Top 0.254: v54.55,54.35 54.55,42 55.05,41.5 55.05,30.3 v57.3,28.05
  Bottom 0.254: IC3.1 54.53,54.37 v54.55,54.35 56.05,52.85 R28.1 | v57.3,28.05 67.13,28.05 J1.AP-EINT1
L+OUT  (via drill 0.3)
  Top 0.254: PAM1.1 54.18,38.77 54.6,38.35 54.6,15.65 v56.05,14.2
  Bottom 0.254: v56.05,14.2 82.99,14.2 L+.1
L-OUT  (via drill 0.3)
  Top 0.254: v57.1,9.4 54,12.5 54,36.05 53.82,36.23 PAM1.3
  Bottom 0.254: L-.1 80.45,8.9 57.6,8.9 v57.1,9.4
L_TRIGGER  (via drill 0.3)
  Top 0.254: v9.6,60.35 7.75,60.35 7.05,59.65 L_BUTTONS.10
  Bottom 0.254: IC3.8 30.77,60.92 28.65,58.8 11.15,58.8 v9.6,60.35 8.75,61.2 R19.1
LCD_D3  (via drill 0.3)
  Top 0.254: DISP_DATA.24 30.75,35.15 v29.95,34.35
  Bottom 0.254: v29.95,34.35 30.3,34.7 33.75,34.7 35.4,33.05 37.63,33.05 J1.LCD-D3
LCD_D4  (via drill 0.3)
  Top 0.254: DISP_DATA.25 31.25,34.45 v30.85,34.05
  Bottom 0.254: v30.85,34.05 30.85,33.2 31,33.05 31.63,33.05 J1.LCD-D4
LCD_D5  (via drill 0.3)
  Top 0.254: DISP_DATA.26 v31.75,32.05
  Bottom 0.254: v31.75,32.05 34.6,32.05 36.13,30.52 J1.LCD-D5
LCD_D6  (via drill 0.3)
  Top 0.254: DISP_DATA.27 32.25,42.5 32.9,41.85 32.9,31.95 v32.35,31.4
  Bottom 0.254: v32.35,31.4 31.64,30.69 J1.LCD-D6
LCD_D7  (via drill 0.3)
  Top 0.254: DISP_DATA.28 32.75,42.7 33.45,42 33.45,29.6 v33.05,29.2
  Bottom 0.254: v33.05,29.2 35.1,29.2 36.32,27.98 J1.LCD-D7
LCD_D10  (via drill 0.3)
  Top 0.254: DISP_DATA.15 26.25,28.2 v26,27.95
  Bottom 0.254: v26,27.95 31.61,27.95 J1.LCD-D10
LCD_D11  (via drill 0.3)
  Top 0.254: DISP_DATA.16 26.75,26.85 v26.5,26.6
  Bottom 0.254: v26.5,26.6 34.15,26.6 35.3,25.45 J1.LCD-D11
LCD_D12  (via drill 0.3)
  Top 0.254: DISP_DATA.17 27.25,25.7 v27,25.45
  Bottom 0.254: v27,25.45 J1.LCD-D12
LCD_D13  (via drill 0.3)
  Top 0.254: DISP_DATA.18 27.75,24.55 v27.5,24.3
  Bottom 0.254: v27.5,24.3 34.1,24.3 35.5,22.9 J1.LCD-D13
LCD_D14  (via drill 0.3)
  Top 0.254: DISP_DATA.19 28.25,23.5 v28.85,22.9
  Bottom 0.254: v28.85,22.9 J1.LCD-D14
LCD_D15  (via drill 0.3)
  Top 0.254: DISP_DATA.20 28.75,24 v31.15,21.6
  Bottom 0.254: v31.15,21.6 31.4,21.85 34.45,21.85 35.94,20.36 J1.LCD-D15
LCD_D19  (via drill 0.3)
  Top 0.254: DISP_DATA.8 22.75,23.25 v22.4,22.9
  Bottom 0.254: J1.LCD-D19 37.64,18.21 37.15,18.7 29.35,18.7 27.3,20.75 23.55,20.75 22.4,21.9 v22.4,22.9
LCD_D20  (via drill 0.3)
  Top 0.254: DISP_DATA.9 23.25,22.75 22.55,22.05 22.55,20.7 v23,20.25
  Bottom 0.254: v23,20.25 26.8,20.25 29.23,17.82 J1.LCD-D20
LCD_D21  (via drill 0.3)
  Top 0.254: DISP_DATA.10 23.75,22.1 v23.45,21.8
  Bottom 0.254: J1.LCD-D21 37.66,15.3 40.75,15.3 41.3,15.85 41.3,18.75 40.65,19.4 29.4,19.4 27,21.8 v23.45,21.8
LCD_D22  (via drill 0.3)
  Top 0.254: DISP_DATA.11 24.25,19.85 v23.85,19.45
  Bottom 0.254: v23.85,19.45 26.6,19.45 26.85,19.2 26.85,15.8 27.3,15.35 31.57,15.35 J1.LCD-D22
LCD_D23  (via drill 0.3)
  Top 0.254: DISP_DATA.12 24.75,13 v26,11.75
  Bottom 0.254: v26,11.75 35.1,11.75 36.1,12.75 J1.LCD-D23
LEFT  (via drill 0.3)
  Top 0.254: L_BUTTONS.8 7.95,58.65 8.4,59.1 9.25,59.1 v9.35,59
  Bottom 0.254: IC3.7 30.88,60.27 28.9,58.3 10.05,58.3 9.7,58.65 v9.35,59 9.2,59.15 R20.1
MUTE  (via drill 0.3)
  Top 0.254: R_BUTTONS.6 77.25,58.65 72.4,63.5 v72.4,63.95
  Bottom 0.254: v72.4,63.95 71.97,63.52 66.85,63.52 | 66.85,63.52 IC3.13 | R14.1 66.7,65.5 66.8,65.4 66.8,63.58 66.85,63.52
N$1
  Bottom 0.254: U$27.4 5.31,22.03 7.67,22.03 8.32,21.38 8.32,16.79 9.03,16.08 IC1.4
N$27
  Bottom 0.254: 21.25,16.5 20.65,15.9 20.65,9.35 21.6,8.4 27.25,8.4
N$38
  Top 0.254: PAM1.8 50.78,29.88 50.1,29.2 49.18,29.2 C6.1
N$41
  Top 0.254: R4.1 47.28,30.83 C14.1
N$43
  Top 0.254: C13.1 65.33,31.18 R5.1
PWM  (via drill 0.3)
  Top 0.254: v14.15,16.95 v14.15,36.3
  Bottom 0.254: IC1.2 13.94,16.74 v14.15,16.95 | v14.15,36.3 14.7,36.85 34.75,36.85 35.95,35.65 37.59,35.65 J1.PWM0
PWR_ON  (via drill 0.3)
  Top 0.254: R_BUTTONS.12 v80.25,52.45
  Bottom 0.254: J1.PWRON 37.7,45.7 55.8,45.7 62.55,52.45 62.9,52.45 | R25.1 62.9,52.45 | 62.9,52.45 75.5,52.45 75.8,52.15 76.75,52.15 77.05,52.45 v80.25,52.45
R+OUT  (via drill 0.3)
  Top 0.254: PAM1.16 56.92,38.77 v56.9,38.75 | v44.15,37.45 42.6,35.9 42.6,11.55 41.4,10.35 6.96,10.35 R+.1
  Bottom 0.254: v56.9,38.75 45.45,38.75 v44.15,37.45
R-OUT  (via drill 0.3)
  Top 0.254: v44.2,36.25 43.25,35.3 43.25,11.4 41.65,9.8 8.4,9.8 R-.1 | v56.9,36.25 58.69,36.25 PAM1.14
  Bottom 0.254: v44.2,36.25 v56.9,36.25
R_TRIGGER  (via drill 0.3)
  Top 0.254: v83.6,65 84.3,64.3 84.3,59.05 86.25,57.1 R_BUTTONS.24
  Bottom 0.254: IC3.14 73.42,62.88 74.2,63.65 75.8,63.65 76.5,64.35 76.5,64.95 R13.1 76.65,65 v83.6,65
RIGHT  (via drill 0.3)
  Top 0.254: v8.95,54.85 7.55,54.85 6.75,55.65 L_BUTTONS.2
  Bottom 0.254: IC3.4 31.23,58.33 29.7,56.8 10.9,56.8 v8.95,54.85 8.95,53.9 8.05,53 R23.1
SDIO_CARD
  Bottom 0.254: SDIO.9 46.61,26.06 47.35,26.8 69.4,26.8 70.6,28 73.18,28 J1.AP-EINT3
SDIO_CLK
  Bottom 0.254: SDIO.5 51.01,13.89 53.1,11.8 69.55,11.8 70.45,12.7 73.16,12.7 J1.CSID5
SDIO_CMD
  Bottom 0.254: SDIO.3 53.21,14.49 54.96,12.74 J1.CISD4
SDIO_DAT0
  Bottom 0.254: SDIO.7 48.81,23.71 49.25,24.15 56.5,24.15 57,23.65 57,18.6 57.75,17.85 67.17,17.85 J1.CSID0
SDIO_DAT1
  Bottom 0.254: SDIO.8 47.71,24.36 48.25,24.9 56.75,24.9 57.5,24.15 57.5,19.85 58.25,19.1 69.3,19.1 70.6,17.8 73.18,17.8 J1.CSID1
SDIO_DAT2
  Bottom 0.254: SDIO.1 55.41,16.69 56.8,15.3 66.35,15.3 66.45,15.2 67.12,15.2 J1.CSID2
SDIO_DAT3
  Bottom 0.254: SDIO.2 54.31,23.21 54.75,23.65 55.9,23.65 56.35,23.2 56.35,17.9 57.6,16.65 69.15,16.65 70.5,15.3 73.18,15.3 J1.CSID3
SELECT  (via drill 0.3)
  Top 0.254: R_BUTTONS.7 77.75,58.8 74.35,62.2 v74.35,62.5 | v59.25,62.55 56.7,62.55 R11.1
  Bottom 0.254: v74.35,62.5 74.08,62.23 IC3.15 59.58,62.23 v59.25,62.55
SQUARE  (via drill 0.3)
  Top 0.254: R_BUTTONS.18 83.25,56.3 81.25,58.3 79.5,58.3 77.1,60.7 v77.1,60.95 | R2.1 59.55,61.05 v59.4,60.9
  Bottom 0.254: v77.1,60.95 77.08,60.92 IC3.17 59.42,60.92 v59.4,60.9
START  (via drill 0.3)
  Top 0.254: v78.5,57.8 78.25,57.55 R_BUTTONS.8 | v56.65,56.7 56.65,56 56.25,55.6 51.55,55.6 49.25,57.9 R10.1
  Bottom 0.254: v78.5,57.8 77.33,58.98 IC3.20 58.92,58.98 v56.65,56.7
TRIANGE  (via drill 0.3)
  Top 0.254: v82.65,57.85 83.75,56.75 R_BUTTONS.19 | v55.8,58.15 53.4,58.15 R3.1
  Bottom 0.254: v82.65,57.85 81.8,58.7 79.65,58.7 78.08,60.27 IC3.18 57.92,60.27 v55.8,58.15
UP  (via drill 0.3)
  Top 0.254: L_BUTTONS.4 7.7,56.65 v8.25,57.2
  Bottom 0.254: R21.1 7.15,57.2 v8.25,57.2 8.85,57.8 29.15,57.8 30.98,59.62 IC3.6
VBAT_EXT  (via drill 0.3)
  Top 0.254: v55.55,48.3 55.55,45.8 55.2,45.45 55.2,42.9 55.5,42.6 BAT.1
  Bottom 0.254: J1.BAT 53.5,48.3 v55.55,48.3
VCC3V3  (via drill 0.3)
  Top 0.254: DISP_DATA.4 20.75,49.45 | 20.75,49.45 22.25,50.95 | 22.25,50.95 v28.15,50.95 | DISP_DATA.3 20.25,48.95 20.75,49.45 | v24.75,11.95 15.6,11.95 15.15,12.4 v15.15,14.25 v15.15,17 v15.15,18 15.15,35.5 | 15.15,35.5 15.15,48.45 17.65,50.95 22.25,50.95 | v15.7,35.5 15.15,35.5 | v40.8,20.6 40.8,37.15 42.55,38.9 42.55,48.7 42.48,48.77 | 42.48,48.77 v41.5,49.75 | R15.2 45.09,62.1 | 45.09,62.1 45.08,60 | 45.08,60 45.08,57.75 | 45.08,57.75 45.05,51.35 42.65,48.95 | 42.65,48.95 42.48,48.77 | v60.2,53.55 60.2,51.25 v59.65,50.7 | C9.1 42.69,48.91 42.65,48.95 | v52.1,19.3 v50.15,19.3 | R15.2 45.1,65.6 45.4,65.9 71.85,65.9 v72.25,65.5 | R1.2 R2.2 56.2,59.15 R11.2 53.8,59.65 R3.2 R9.2 R10.2 47.95,58.8 47.95,58.5 47.2,57.75 45.08,57.75 | R15.2 45.05,64.2 | R17.2 45.09,62.1 | R16.2 45.08,60.08 45.08,60
  Bottom 0.254: IC2.5 23.86,12.84 v24.75,11.95 | IC2.11 15.29,14.11 v15.15,14.25 | IC2.13 15.5,16.65 v15.15,17 | IC2.14 15.23,17.92 v15.15,18 14.75,18.4 9.4,18.4 9.2,18.2 9.2,17.95 9.76,17.39 IC1.5 | R12.2 v15.7,35.5 | R19.2 R20.2 R21.2 R22.2 R23.2 5.2,52.95 5.2,51.5 5.45,51.25 13.15,51.25 13.45,50.95 v28.15,50.95 30.85,50.95 31.05,50.75 31.55,50.75 J1.VCC3V3@2 32.73,49.75 v41.5,49.75 58.7,49.75 v59.65,50.7 | 58.7,54.5 58.95,54.5 C16.2 | C16.2 58.89,54.9 IC3.24 | SDIO.4 v52.11,19.31 v52.1,19.3 | R28.2 59.5,52.85 v60.2,53.55 | v60.2,53.55 58.85,54.9 C16.2 | R25.2 61.15,54.5 v60.2,53.55 | v50.15,19.3 42.1,19.3 v40.8,20.6 | C1.1 14.9,14 v15.15,14.25 | R24.2 80.35,53.85 81.5,55 85.4,55 | 85.4,55 87.1,55 87.6,55.5 87.6,56.2 84.65,59.15 84.65,64.95 83.35,66.25 74.95,66.25 74.7,66 R13.2 74.25,65.5 v72.25,65.5 R14.2 | R26.2 R27.2 85.35,54.95 85.4,55 | IC2.9 15.98,11.57 15.15,12.4 v15.15,14.25
VCC3V3_2
  Bottom 0.254: J1.VCC3V3@1 62.61,45.76 62.25,45.4 62.25,43.45 SJ3.1
VCC5V  (via drill 0.3)
  Top 0.254: R_BUTTONS.22 85.25,56.3 v85.55,56.6 | 36.55,50.05 C10.1 36.25,50.05 | 36.24,52.11 C7.1 36.12,52.1 | DISP_DATA.35 36.25,49 | 36.25,49 36.25,50.05 | 36.25,50.05 36.25,51.98 36.12,52.1 | DISP_DATA.36 36.75,48.5 36.25,49 | 36.12,52.1 v39.95,52.1 | v48.15,52.05 v48.15,43.15
  Top 0.406: v70.5,55.3 66.55,51.35 66.55,44.65 65.85,43.95 v57.1,43.95 | v43.95,43.15 43.95,38.5 41.9,36.45 41.9,11.85 41.05,11 v4.6,11
  Bottom 0.254: v85.55,56.6 84.87,55.92 J1.VCC-5V@2 73.16,55.96 71.16,55.96 v70.5,55.3 | v39.95,52.1 48.1,52.1 v48.15,52.05 | SJ3.3 48.8,40.35 48.15,41 v48.15,43.15
  Bottom 0.406: v57.1,43.95 56.3,43.15 v48.15,43.15 v43.95,43.15
  Bottom 0.61: U$27.6 2.24,24.89 1.72,25.41
  Bottom 0.813: L2.P$2 2.73,32.28 1.68,31.23 1.72,25.41 1.72,20.8 | 1.72,20.8 1.72,18.3 | 1.72,18.3 1.72,13.88 v4.6,11 | C4.1 2,20.52 1.72,20.8 | C2.1 1.75,18.32 1.72,18.3
VOL+  (via drill 0.3)
  Top 0.254: R_BUTTONS.4 76.25,58.3 70.75,63.8 51.2,63.8 50.85,64.15 49.8,64.15 v49.05,63.4 | 48.95,63.5 v49.05,63.4 | R17.1 47.8,62.15 v49.05,63.4
  Bottom 0.254: v49.05,63.4 49.1,62.05 49.58,61.58 IC3.9
VOL-  (via drill 0.3)
  Top 0.254: R_BUTTONS.3 75.75,58.15 70.6,63.3 v50.3,63.3 50,63.3 47,60.3 R16.1
  Bottom 0.254: v50.3,63.3 50.3,62.55 50.6,62.25 54.51,62.25 IC3.10
VOUT  (via drill 0.3)
  Top 0.406: v41.9,55.95 41.9,52.05 40.45,50.6 40.45,46.3 39,44.85 39,14.6 v40.65,12.95 | v62.7,10.8 72.35,10.8 79.6,18.05 84.45,18.05 POWERIN.1
  Bottom 0.254: 41.87,55.92 v41.9,55.95
  Bottom 0.406: J1.CHG-IN 41.87,55.92 | v40.65,12.95 49.05,12.95 51.1,10.9 62.6,10.9 v62.7,10.8
VREG_OUTPUT
  Bottom 0.61: U$27.1 7.96,24.89 8.42,25.35 8.38,31.55 L2.P$1
  Bottom 1.27: L2.P$1 7.65,37.5 D2.A
VSYNC
  Bottom 0.254: J1.LCD-VSYNC 28.55,10.2 27.25,8.9 21.7,8.9 21.15,9.45 21.15,15 21.5,15.35 22.83,15.35 IC2.3
X  (via drill 0.3)
  Top 0.254: R_BUTTONS.17 82.75,56.2 81.1,57.85 79.35,57.85 75.9,61.3 v75.9,61.8 | R1.1 58.05,61.45 v58.5,61.9
  Bottom 0.254: v75.9,61.8 75.67,61.58 IC3.16 59.42,61.58 59.1,61.9 v58.5,61.9

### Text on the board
tNames: 1 | 40 | CSP I | CHIPDIPSHOP
bNames: CHIPDIPSHOP | CSP I | v1 / JKW

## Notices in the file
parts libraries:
JKW_CHIP: License : http://creativecommons.org/licenses/by-sa/3.0
(Creative Commons 3.0)
